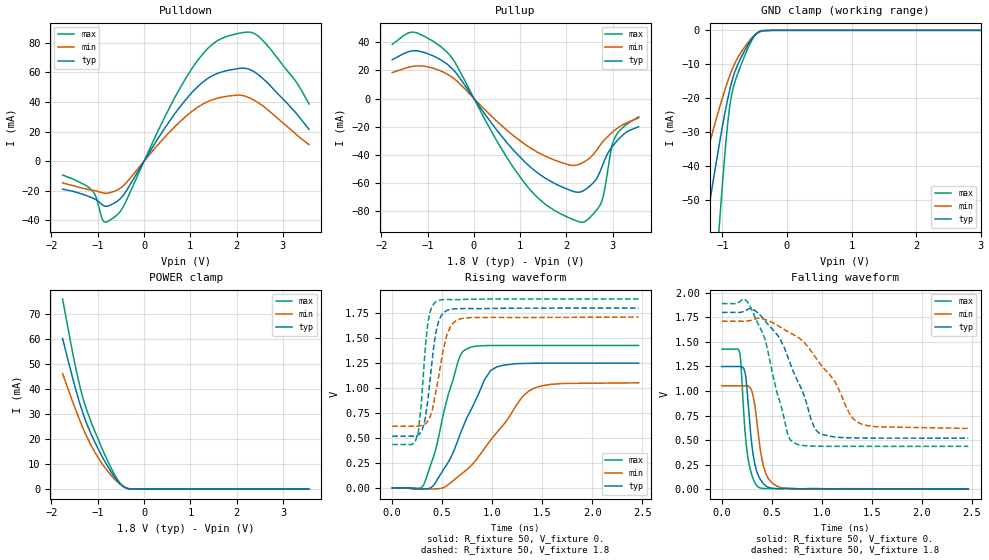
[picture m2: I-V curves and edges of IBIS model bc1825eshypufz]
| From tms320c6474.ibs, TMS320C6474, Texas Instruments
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|   MODEL bc1825eshypufz
[Model] bc1825eshypufz
Model_type I/O
|C_comp_off 928.861f 857.257f 967.727f
|C_comp_on 803.685f 724.633f 843.474f
C_comp 866.273f 790.945f 905.6f
|Rth_i 107.818Meg 12.199Meg 895.331Meg
|Rth_r 23.374 32.235 17.647
|Rth_f 21.657 29.516 16.232
Vinl = 0.630
Vinh = 1.170
Vmeas = 0.9
Cref = 5pF
[Model Spec]
||   Typ   Min   Max
S_overshoot_high   2.100   2.010   2.190
Vinh   1.170   1.111   1.229
Vmeas   0.900   0.855   0.945
Vinl   0.630   0.599   0.662
S_overshoot_low   -0.300  -0.300  -0.300
[Receiver Thresholds]
Vth   = 0.900V
Vth_min = 0.855V
Vth_max = 0.945V
Vinh_ac = +270mV   || Undefined so set to Vinh_dc level
Vinh_dc = +270mV
Vinl_dc = -270mV
Vinl_ac = -270mV   || Undefined so set to Vinl_dc level
Tslew_ac = 5.0ns   || Undefined in specification - set to large value
|| Pointer to HSPICE models:
|ff ti_bc1825eshypufz.mod ti_bc1825eshypufz_ff
|tt ti_bc1825eshypufz.mod ti_bc1825eshypufz_tt
|ss ti_bc1825eshypufz.mod ti_bc1825eshypufz_ss
|| Spice2IBIS controls:
|View_IV No
[Temperature Range]  25   105   -40
|corevdd   1.100  1.045  1.155
[Voltage Range]   1.8   1.71   1.89
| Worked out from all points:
|   slope of the pulldown table from 0 to 0.27 V, typ, clamps not added: 19.6 ohm
|   slope of the pullup table from 0 to 0.27 V, typ, clamps not added: 21.3 ohm
|   GND clamp passes 1 mA (typ) near -0.48 V on its own axis
|   POWER clamp passes 1 mA (typ) near -0.44 V on its own axis
|   rising waveform, R_fixture 50, V_fixture 0.: 20-80 % time 333ps typ, 475ps min, 221ps max; typ from 0 V to 1.25 V
|   rising waveform, R_fixture 50, V_fixture 1.8: 20-80 % time 93ps typ, 125ps min, 72ps max; typ from 0.519 V to 1.8 V
|   falling waveform, R_fixture 50, V_fixture 0.: 20-80 % time 77.5ps typ, 91.5ps min, 67.8ps max; typ from 1.25 V to 0 V
|   falling waveform, R_fixture 50, V_fixture 1.8: 20-80 % time 299ps typ, 418ps min, 218ps max; typ from 1.8 V to 0.519 V
[Pulldown]
-1.76V    -18.87mA   -14.66mA   -9.328mA
-1.13V    -24.63mA   -19.54mA   -19.47mA
-860.6mV  -30.2mA    -21.62mA   -40.97mA
-607.4mV  -27.67mA   -19.84mA   -36.96mA
-429.7mV  -22.22mA   -16.05mA   -29.68mA
442.9mV   22.09mA    16.07mA    29.55mA
889.9mV   41.15mA    29.87mA    55.34mA
1.364V    55.58mA    40.06mA    75.68mA
1.811V    61.31mA    43.92mA    84.49mA
2.457V    58.72mA    39.72mA    84.66mA
3.238V    34.23mA    19.5mA     55.72mA
3.567V    21.51mA    11.15mA    38.68mA
[Pullup]
-1.767V   27.71mA    18.45mA    38.57mA
-1.309V   34.09mA    23.03mA    47.37mA
-587.2mV  24.73mA    17.54mA    33.27mA
484.6mV   -22.17mA   -15.91mA   -29.71mA
1.109V    -45.58mA   -32.86mA   -60.92mA
1.535V    -56.69mA   -40.98mA   -75.26mA
2.273V    -66.82mA   -46.9mA    -87.88mA
2.58V     -60.11mA   -39.86mA   -82.27mA
2.752V    -49.96mA   -32.1mA    -74.15mA
2.973V    -35.01mA   -24.6mA    -35.25mA
3.059V    -31.45mA   -22.17mA   -27.03mA
3.56V     -20.12mA   -13.86mA   -13.03mA
[GND Clamp]
-1.76V    -120.1mA   -77.08mA   -249.9mA
-1.52V    -90.11mA   -57.65mA   -187.2mA
-1.294V   -62.31mA   -40.14mA   -124.9mA
-1.214V   -52.7mA    -34.31mA   -102.6mA
-1.048V   -33.47mA   -22.94mA   -57.36mA
-934.3mV  -21.71mA   -15.95mA   -30.5mA
-894.4mV  -18.15mA   -13.74mA   -23.47mA
-854.4mV  -15.08mA   -11.75mA   -18.69mA
-787.8mV  -11.24mA   -8.967mA   -14.1mA
-628mV    -5.016mA   -4.163mA   -6.265mA
-441.5mV  -540.3uA   -650.4uA   -459.2uA
3.567V    0A         0A         0A
[Power Clamp]
-1.76V    60.41mA    46.34mA    76.15mA
-1.582V   47.3mA     37.05mA    58.41mA
-1.466V   39.29mA    31.25mA    47.67mA
-1.369V   33.14mA    26.63mA    39.8mA
-1.271V   27.78mA    22.37mA    33.46mA
-1.166V   22.91mA    18.28mA    27.93mA
-1.05V    18.28mA    14.36mA    22.51mA
-774.1mV  8.755mA    6.901mA    10.78mA
-596.5mV  3.873mA    3.258mA    4.507mA
-447.9mV  1.11mA     1.087mA    1.053mA
-252.1mV  23.65uA    39.8uA     15.54uA
3.56V     0A         0A         0A
[Ramp]
dV/dt_r .749/332.594p .632/475.371p .856/221.178p
dV/dt_f .768/299.341p .655/418.146p .873/217.618p
[Rising Waveform]
R_fixture = 50
V_fixture = 0.
0s        0V         1.296uV    0V
315ps     -9.19mV    -6.284mV   33.76mV
430ps     51.48mV    -7.754mV   368.8mV
555ps     249.9mV    29.99mV    913.5mV
675ps     527.1mV    127.8mV    1.312V
725ps     651.5mV    167.1mV    1.38V
985ps     1.175V     480.7mV    1.425V
1.3ns     1.246V     910.2mV    1.426V
1.415ns   1.248V     996.7mV    1.426V
2.465ns   1.249V     1.052V     1.426V
[Rising Waveform]
R_fixture = 50
V_fixture = 1.8
V_fixture_min = 1.71
V_fixture_max = 1.89
0s        519.2mV    618.2mV    435.6mV
195ps     519.1mV    618.4mV    435.9mV
260ps     531.8mV    618.8mV    554.9mV
305ps     599.2mV    627.8mV    1.045V
355ps     868.6mV    669.3mV    1.638V
395ps     1.238V     762.8mV    1.809V
440ps     1.571V     983.4mV    1.866V
545ps     1.774V     1.528V     1.886V
665ps     1.794V     1.686V     1.884V
2.465ns   1.8V       1.71V      1.89V
[Falling Waveform]
R_fixture = 50
V_fixture = 0.
0s        1.249V     1.053V     1.426V
180ps     1.25V      1.053V     1.383V
190ps     1.25V      1.053V     1.292V
230ps     1.195V     1.054V     610.9mV
260ps     912.4mV    1.05V      323.3mV
310ps     366.9mV    958.9mV    113.4mV
365ps     139.7mV    559.7mV    21.81mV
440ps     34.08mV    158.1mV    6.721mV
585ps     5.632mV    17.83mV    4.092mV
2.465ns   43.4uV     187.3uV    780.2nV
[Falling Waveform]
R_fixture = 50
V_fixture = 1.8
V_fixture_min = 1.71
V_fixture_max = 1.89
0s        1.8V       1.71V      1.89V
225ps     1.813V     1.71V      1.934V
285ps     1.838V     1.718V     1.856V
425ps     1.723V     1.73V      1.545V
575ps     1.544V     1.657V     903.6mV
655ps     1.358V     1.607V     574.2mV
715ps     1.197V     1.574V     476.6mV
935ps     608.8mV    1.344V     437.8mV
1.345ns   521.5mV    688mV      435.6mV
2.465ns   519.3mV    618.6mV    435.6mV
